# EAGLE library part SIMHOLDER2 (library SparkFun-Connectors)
Alternate SIM card socket.
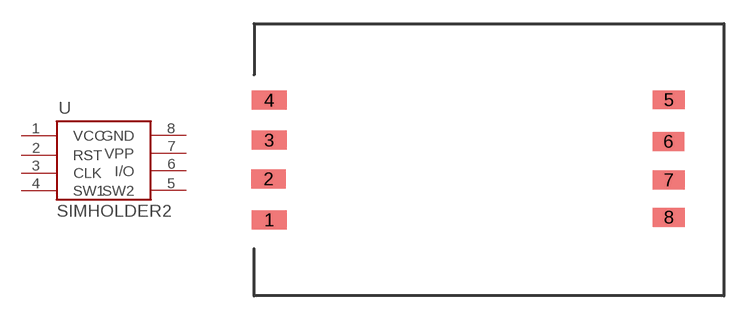
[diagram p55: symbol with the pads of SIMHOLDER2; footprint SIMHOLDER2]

Designator prefix -

## SIMHOLDER2  [SIMHOLDER2]
1  VCC
2  RST
3  CLK
4  SW1
5  SW2
6  I/O
7  VPP
8  GND

## Footprint SIMHOLDER2 (pad centres in mm)
smd 2.2 x 1.2: 1 0.95,4.81; 2 0.91,7.41; 3 0.95,9.86; 4 0.95,12.39
smd 2 x 1.2: 5 26.22,12.42; 6 26.2,9.78; 7 26.22,7.34; 8 26.22,4.98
